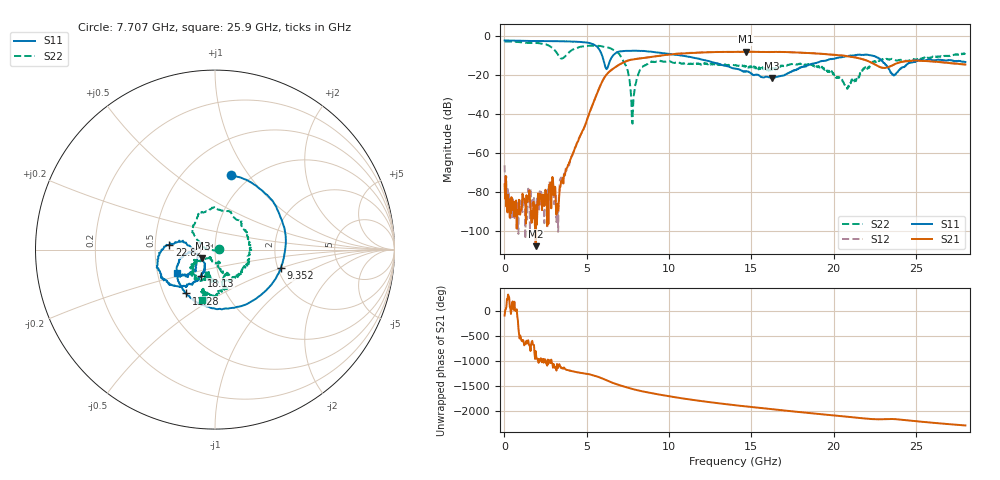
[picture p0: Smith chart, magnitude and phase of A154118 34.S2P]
!  2-Port S-parameters saved by WinCal
! VAR MeasName=S-Parameters (CALIBRATED_DATA) read from VNA (N5230A)
! VAR MeasDate=2015-9-10 14:37:00
! VAR NAME=A154118 34
! VAR FILENAME=A154118 34.S2P
! VAR DATE=2015-9-10 14:37:00
! VAR PHYS_PORTS=1,2
# Hz S DB R 50
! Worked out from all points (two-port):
!   801 points, 10 MHz to 28 GHz, reference 50 ohm
!   highest |S21| = -7.92 dB at 14.67 GHz (marker M1); lowest = -108.1 dB at 1.899 GHz (marker M2)
!   |S21| within 3 dB of the highest: 8.664 GHz to 21.33 GHz (12.66 GHz wide, 84.4 % of centre)
!   lowest |S11| = -21.4 dB at 16.24 GHz (marker M3), VSWR 1.18, Z = 43.3 - j4.19 ohm
!   |S11| at or under -10 dB: 5.936 GHz to 6.589 GHz (653 MHz wide, 10.4 % of centre); 10.83 GHz to 20.93 GHz (10.1 GHz wide, 63.6 % of centre); 22.38 GHz to end of sweep
!   |S22| runs from -45.0 to -2.7 dB; largest |S21 - S12| = 0.0092
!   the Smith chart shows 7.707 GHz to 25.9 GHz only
!   S11 on the Smith chart (normalised r, x): 7.707 GHz: 0.82, +0.82; 9.352 GHz: 2.07, -0.50; 11.28 GHz: 0.65, -0.35; 18.13 GHz: 0.82, -0.25; 22.82 GHz: 0.59, +0.03; 25.9 GHz: 0.63, -0.17
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1e7  -2.15 179.7  -76.22 -83.7  -66.40 120.2  -2.67 179.8
2.899e8  -2.19 175.7  -85.21 -88.6  -83.82 174.2  -2.71 172.9
1.899325e9  -2.41 155.0  -108.05 -78.0  -89.52 -41.9  -3.43 131.6
3.193862e9  -2.51 134.9  -87.27 26.0  -88.21 79.0  -8.71 25.6
3.753662e9  -2.59 123.8  -68.30 -91.3  -69.29 -88.6  -9.81 -108.7
4.698325e9  -3.01 98.2  -49.60 -155.8  -49.59 -157.8  -5.29 166.4
6.097825e9  -14.86 -53.0  -20.89 72.6  -20.83 72.5  -5.56 103.5
6.937525e9  -7.91 118.5  -14.78 -32.9  -14.75 -33.2  -8.82 54.6
7.70725e9  -7.48 78.0  -12.06 -109.6  -12.04 -109.8  -33.15 3.1
8.302038e9  -7.55 48.0  -11.34 -157.4  -11.33 -157.5  -16.52 142.8
9.351662e9  -8.40 -15.9  -10.18 136.0  -10.09 136.0  -12.61 94.1
1.127598e10  -10.67 -123.4  -8.61 34.5  -8.53 33.6  -14.03 15.5
1.4005e10  -16.60 -174.7  -8.01 -79.9  -8.04 -80.5  -14.93 -87.7
1.466976e10  -18.26 -176.9  -7.92 -104.8  -7.90 -105.2  -15.30 -96.4
1.62442e10  -21.45 -145.5  -8.09 -159.7  -8.07 -160.2  -17.34 -106.7
1.813352e10  -15.68 -117.8  -8.54 136.0  -8.49 135.4  -14.38 -125.8
1.869332e10  -14.11 -119.3  -8.71 117.9  -8.72 117.5  -14.50 -131.7
2.079258e10  -10.26 -139.5  -10.24 49.8  -10.14 49.1  -25.98 -116.6
2.282185e10  -11.85 174.1  -15.87 -1.4  -15.86 -2.7  -12.05 -85.6
2.334666e10  -16.87 171.1  -15.74 4.9  -15.79 4.1  -12.00 -96.5
2.590075e10  -12.03 -148.8  -12.92 -67.8  -12.96 -69.3  -10.84 -104.3
2.8e10  -13.29 -155.1  -14.53 -125.2  -14.58 -126.1  -8.61 -113.0
